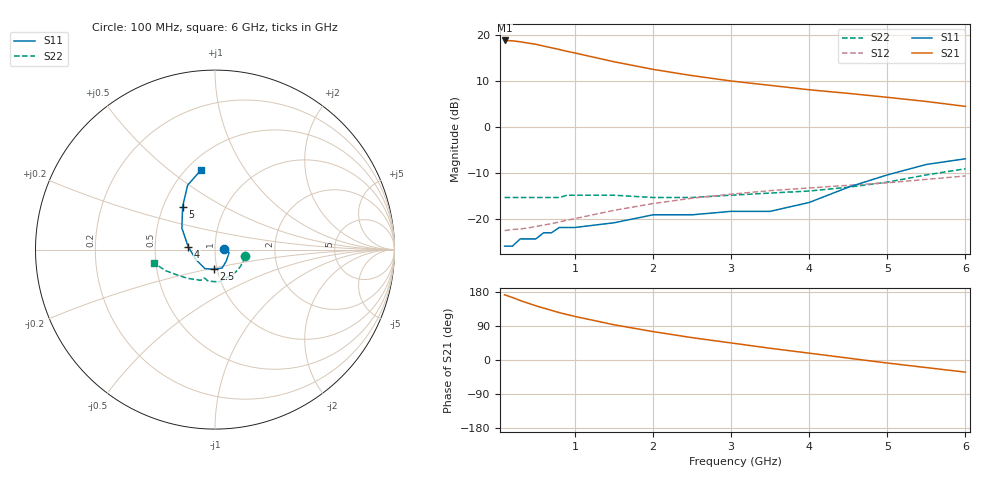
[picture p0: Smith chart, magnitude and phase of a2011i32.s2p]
!  MSA-2011 S PARAMETERS
!  Id = 32 mA  LAST UPDATED 06-27-94
# ghz s ma r 50
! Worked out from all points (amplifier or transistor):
!   20 points, 100 MHz to 6 GHz, reference 50 ohm
!   highest |S21| = 18.9 dB at 100 MHz (marker M1)
!   |S21| within 3 dB of that: start of sweep to 1.069 GHz
!   unconditionally stable (mu >= 1): start of sweep to 5.087 GHz
!   at 400 MHz: K = 1.08, MAG = 18.5 dB, |S12| = -22.0 dB
!   at 1.5 GHz: K = 1.07, MAG = 14.6 dB, |S12| = -18.2 dB
!   at 6 GHz: K = 0.85, MSG = 7.6 dB, |S12| = -10.7 dB
!   S11 on the Smith chart (normalised r, x): 100 MHz: 1.10, +0.01; 2.5 GHz: 0.97, -0.21; 4 GHz: 0.74, +0.02; 5 GHz: 0.63, +0.33; 6 GHz: 0.59, +0.65
0.1  0.05 7.0  8.81 172.0  0.074 4.0  0.17 -13.0
0.2  0.05 9.0  8.73 165.0  0.076 8.0  0.17 -23.0
0.3  0.06 3.0  8.52 157.0  0.077 11.0  0.17 -34.0
0.4  0.06 1.0  8.25 150.0  0.079 15.0  0.17 -43.0
0.5  0.06 0.0  8 143.0  0.082 17.0  0.17 -52.0
0.6  0.07 -5.0  7.65 137.0  0.085 20.0  0.17 -61.0
0.7  0.07 -8.0  7.33 131.0  0.088 22.0  0.17 -68.0
0.8  0.08 -12.0  7.02 125.0  0.092 24.0  0.17 -74.0
0.9  0.08 -18.0  6.7 120.0  0.096 26.0  0.18 -80.0
1  0.08 -22.0  6.43 115.0  0.1 28.0  0.18 -85.0
1.5  0.09 -46.0  5.16 93.0  0.123 31.0  0.18 -102.0
2  0.11 -69.0  4.26 75.0  0.146 31.0  0.17 -109.0
2.5  0.11 -93.0  3.64 59.0  0.167 29.0  0.17 -111.0
3  0.12 -118.0  3.18 45.0  0.185 26.0  0.18 -112.0
3.5  0.12 -152.0  2.85 31.0  0.202 24.0  0.19 -116.0
4  0.15 174.0  2.55 18.0  0.216 21.0  0.2 -124.0
4.5  0.22 147.0  2.33 5.0  0.231 19.0  0.22 -133.0
5  0.3 127.0  2.11 -8.0  0.246 17.0  0.25 -145.0
5.5  0.39 113.0  1.9 -20.0  0.268 14.0  0.3 -157.0
6  0.45 100.0  1.68 -32.0  0.292 10.0  0.35 -168.0
